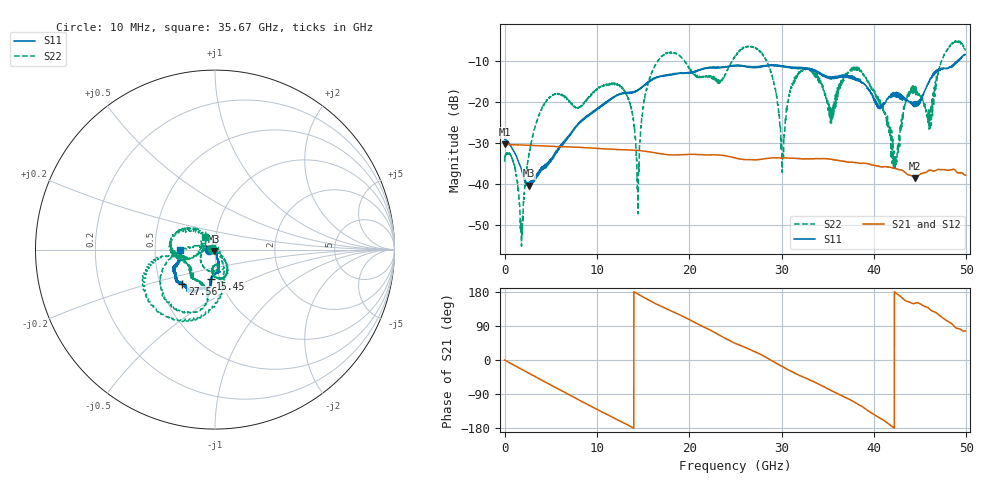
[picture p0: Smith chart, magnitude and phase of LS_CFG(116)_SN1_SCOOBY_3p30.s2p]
!Keysight Technologies,N5245B,MY58422026,A.13.80.08
!Date: Friday, March 20, 2020 00:03:37
!Correction: S11(Full 2 Port(1,2))
!S21(Full 2 Port(1,2))
!S12(Full 2 Port(1,2))
!S22(Full 2 Port(1,2))
!S2P File: Measurements: S11, S21, S12, S22:
# Hz S DB R 50.0
!freq dBS11 angS11 dBS21 angS21 dBS12 angS12 dBS22 angS22
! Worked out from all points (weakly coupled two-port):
!   4991 points, 10 MHz to 49.91 GHz, reference 50 ohm
!   highest |S21| = -30.47 dB at 20 MHz (marker M1); lowest = -38.7 dB at 44.45 GHz (marker M2)
!   lowest |S11| = -40.5 dB at 2.63 GHz (marker M3), VSWR 1.02, Z = 49.5 - j0.807 ohm
!   |S11| at or under -10 dB: start of sweep to 49.12 GHz; 49.17535 GHz to 49.21978 GHz (44.42 MHz wide, 0.0903 % of centre)
!   |S22| runs from -55.3 to -5.1 dB; largest |S21 - S12| = 0.00029
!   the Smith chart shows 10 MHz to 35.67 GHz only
!   S11 on the Smith chart (normalised r, x): 10 MHz: 0.93, -0.01; 15.45 GHz: 0.90, -0.31; 27.56 GHz: 0.65, -0.27; 35.67 GHz: 0.68, -0.00
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1e7  -29.21 -175.5  -30.49 -0.2  -30.46 -0.3  -34.69 177.0
2e7  -29.13 -178.9  -30.47 -0.3  -30.45 -0.4  -33.43 -178.9
1.83e9  -36.50 -161.2  -30.60 -24.3  -30.59 -24.3  -54.89 -16.3
2.63e9  -40.51 -120.2  -30.68 -34.8  -30.66 -34.8  -33.09 131.8
4.78e9  -34.62 -67.4  -30.88 -62.9  -30.87 -62.9  -19.22 -132.5
8.33e9  -24.90 -74.8  -31.21 -109.1  -31.20 -109.0  -21.05 -92.6
1.276e10  -18.05 -78.1  -31.76 -164.1  -31.75 -164.0  -16.74 -63.0
1.445e10  -17.29 -90.4  -31.93 174.0  -31.92 174.1  -45.86 -110.0
1.545e10  -15.56 -98.3  -32.21 160.5  -32.20 160.5  -16.13 175.7
1.665e10  -14.05 -97.6  -32.65 145.1  -32.64 145.2  -9.97 -157.3
2.496e10  -11.29 -123.4  -33.73 44.2  -33.72 44.3  -9.08 -167.9
2.756e10  -11.58 -133.5  -34.14 16.8  -34.14 17.0  -7.73 -110.0
3.011e10  -11.54 -143.7  -33.81 -17.4  -33.80 -17.1  -34.48 16.1
3.116e10  -11.70 -148.5  -33.83 -31.2  -33.84 -30.9  -15.62 140.1
3.328e10  -12.21 -158.5  -33.97 -55.3  -33.96 -54.8  -12.35 -175.2
3.567e10  -14.31 -179.8  -34.21 -84.0  -34.13 -83.6  -20.95 127.9
3.816e10  -14.92 173.2  -34.93 -115.0  -34.87 -115.2  -11.57 -174.5
4.16e10  -18.86 105.0  -35.98 -168.7  -36.02 -168.7  -25.74 67.7
4.233e10  -18.06 104.2  -36.33 178.0  -36.34 177.9  -33.62 165.9
4.445e10  -20.53 54.1  -38.73 149.9  -38.73 150.1  -16.85 -9.9
4.6e10  -15.33 9.4  -36.72 135.2  -36.74 135.3  -24.49 112.2
4.991e10  -8.53 -12.4  -37.96 76.6  -38.00 76.5  -7.38 -14.6
